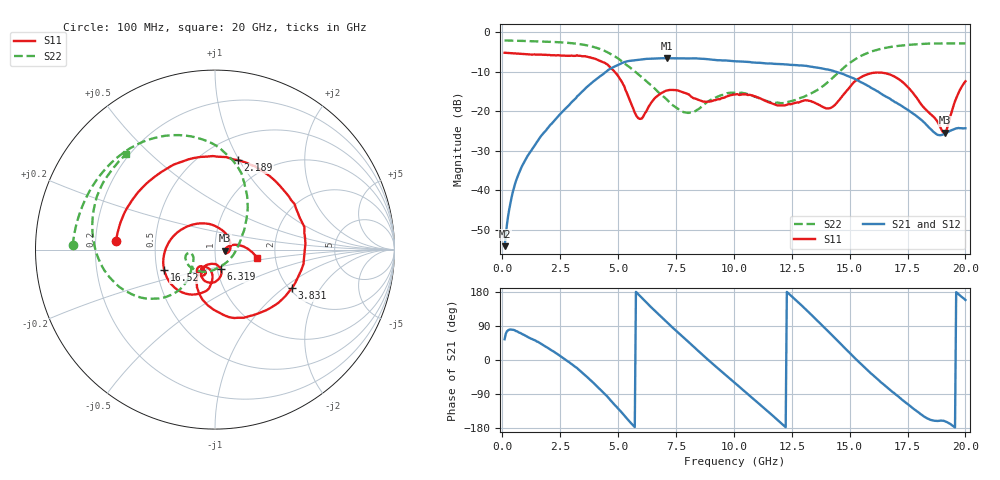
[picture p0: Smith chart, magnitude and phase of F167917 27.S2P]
!  2-Port S-parameters saved by WinCal
! VAR MeasName=S-Parameters (CALIBRATED_DATA) read from VNA (N5242A)
! VAR MeasDate=2016-11-22 9:01:02
! VAR NAME=F167917 27
! VAR FILENAME=F167917 27.S2P
! VAR DATE=2016-11-22 9:01:02
! VAR PHYS_PORTS=1,2
# Hz S DB R 50
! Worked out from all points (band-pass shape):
!   401 points, 100 MHz to 20 GHz, reference 50 ohm
!   highest |S21| = -6.53 dB at 7.115 GHz (marker M1); lowest = -54.2 dB at 100 MHz (marker M2)
!   |S21| within 3 dB of the highest: 4.573 GHz to 14.15 GHz (9.579 GHz wide, 102 % of centre)
!   lowest |S11| = -25.5 dB at 19.1 GHz (marker M3), VSWR 1.11, Z = 55.6 - j0.621 ohm
!   |S11| at or under -10 dB: 4.857 GHz to end of sweep
!   |S22| runs from -20.4 to -2.0 dB; largest |S21 - S12| = 0.0032
!   S11 on the Smith chart (normalised r, x): 100 MHz: 0.29, +0.04; 2.189 GHz: 0.73, +0.99; 3.831 GHz: 2.08, -1.15; 6.319 GHz: 1.04, -0.23; 16.52 GHz: 0.55, -0.14; 20 GHz: 1.61, -0.17
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1e8  -5.15 175.2  -54.21 54.8  -54.11 56.7  -2.02 178.3
7.4675e8  -5.42 145.5  -35.31 71.9  -35.25 71.5  -2.12 167.9
2.1895e9  -5.77 75.6  -22.76 23.4  -22.77 23.2  -2.40 144.0
3.43325e9  -6.01 0.7  -15.08 -32.4  -15.09 -32.3  -3.04 117.6
3.83125e9  -6.37 -26.3  -12.93 -54.3  -12.92 -54.2  -3.50 107.3
4.9755e9  -10.83 -104.0  -8.31 -126.4  -8.28 -126.5  -6.49 74.2
5.871e9  -21.74 -104.3  -6.93 173.6  -6.91 173.5  -10.57 52.0
6.31875e9  -18.84 -73.6  -6.69 145.8  -6.68 145.8  -12.85 41.2
6.7665e9  -15.81 -81.9  -6.55 119.4  -6.54 119.4  -15.29 28.0
7.11475e9  -14.72 -93.1  -6.53 99.2  -6.53 99.3  -17.10 14.1
8.60725e9  -17.43 -118.6  -6.66 16.0  -6.64 16.0  -18.78 -94.7
1.005e10  -15.74 -118.2  -7.29 -60.9  -7.28 -60.8  -15.29 -156.6
1.09455e10  -16.27 -131.2  -7.66 -108.1  -7.61 -108.1  -16.37 -172.4
1.19405e10  -18.50 -127.4  -8.00 -160.7  -7.96 -160.9  -17.83 -164.3
1.338325e10  -17.57 -125.1  -8.70 117.2  -8.68 117.4  -15.31 -140.1
1.417925e10  -19.15 -108.7  -9.55 69.3  -9.56 69.5  -11.97 -131.4
1.487575e10  -14.77 -95.8  -10.95 26.3  -10.88 26.6  -8.30 -136.4
1.65175e10  -10.32 -157.9  -16.09 -66.8  -15.96 -67.0  -3.93 -171.6
1.67165e10  -10.62 -168.0  -16.71 -77.3  -16.72 -77.2  -3.72 -175.7
1.776125e10  -15.53 119.3  -20.67 -128.7  -20.60 -128.4  -3.04 165.4
1.91045e10  -25.46 -6.0  -25.69 -161.4  -25.58 -161.1  -2.78 144.6
2e10  -12.38 -11.7  -24.30 158.5  -24.17 159.0  -2.78 133.0
